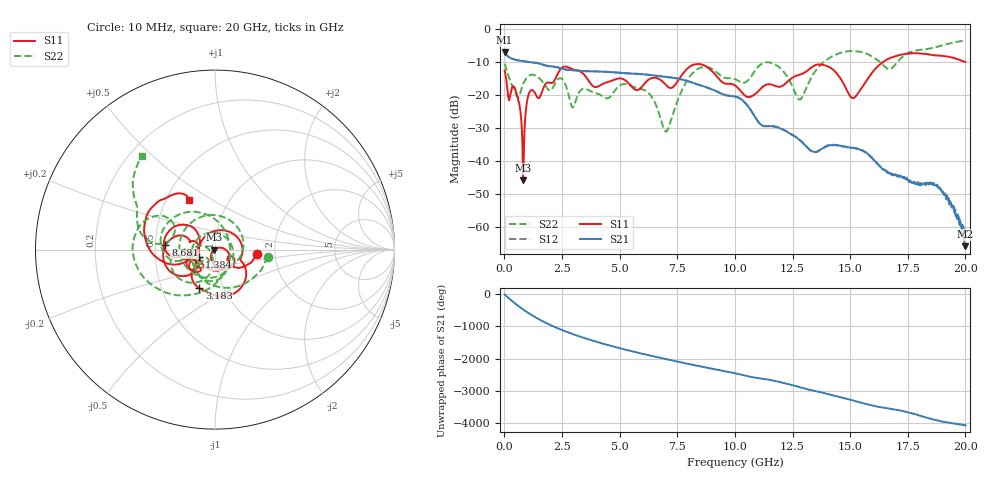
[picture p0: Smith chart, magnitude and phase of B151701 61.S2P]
!  2-Port S-parameters saved by WinCal
! VAR MeasName=S-Parameters (CALIBRATED_DATA) read from VNA (N5244A)
! VAR MeasDate=2015-12-24 19:17:12
! VAR NAME=B151701 61
! VAR FILENAME=B151701 61.S2P
! VAR DATE=2015-12-24 19:17:12
! VAR PHYS_PORTS=1,3
# Hz S DB R 50
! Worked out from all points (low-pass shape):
!   801 points, 10 MHz to 20 GHz, reference 50 ohm
!   highest |S21| = -7.11 dB at 10 MHz (marker M1); lowest = -65.6 dB at 20 GHz (marker M2)
!   |S21| within 3 dB of the highest: start of sweep to 1.075 GHz
!   lowest |S11| = -45.8 dB at 809.6 MHz (marker M3), VSWR 1.01, Z = 49.5 - j0.109 ohm
!   |S11| at or under -10 dB: start of sweep to 16.45 GHz; 19.97441 GHz to end of sweep
!   |S22| runs from -31.1 to -3.6 dB; largest |S21 - S12| = 0.0021
!   S11 on the Smith chart (normalised r, x): 10 MHz: 1.60, -0.09; 1.384 GHz: 0.83, -0.07; 3.183 GHz: 0.77, -0.35; 8.681 GHz: 0.57, +0.03; 20 GHz: 0.65, +0.40
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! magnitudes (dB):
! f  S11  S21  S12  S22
! 10 MHz  -12.6  -7.1  -7.1  -10.6
! 534.7 MHz  -19.8  -9.5  -9.5  -20.3
! 809.6 MHz  -45.8  -9.8  -9.8  -16.8
! 1.059 GHz  -19.7  -10.1  -10.1  -14.3
! 1.384 GHz  -20.2  -10.4  -10.3  -14.3
! 2.959 GHz  -12.3  -12.6  -12.6  -23.8
! 3.183 GHz  -12.7  -12.7  -12.7  -20.1
! 3.358 GHz  -13.2  -12.8  -12.8  -18.3
! 5.357 GHz  -16.3  -13.5  -13.5  -16.8
! 6.682 GHz  -15.2  -14.3  -14.3  -25.0
! 7.056 GHz  -17.3  -14.6  -14.6  -30.9
! 7.906 GHz  -12.3  -15.8  -15.8  -15.9
! 8.681 GHz  -11.1  -17.5  -17.5  -11.6
! 10.01 GHz  -17.1  -20.5  -20.5  -15.2
! 11.58 GHz  -16.9  -29.5  -29.4  -10.4
! 12.8 GHz  -13.9  -33.6  -33.6  -21.4
! 13.35 GHz  -11.5  -37.0  -37.1  -14.3
! 14.23 GHz  -12.2  -35.2  -35.2  -8.4
! 15.13 GHz  -21.0  -36.0  -36.1  -6.8
! 16.68 GHz  -9.1  -43.4  -43.4  -12.3
! 18.83 GHz  -8.1  -47.7  -47.8  -5.4
! 20 GHz  -10.1  -65.6  -64.2  -3.6
